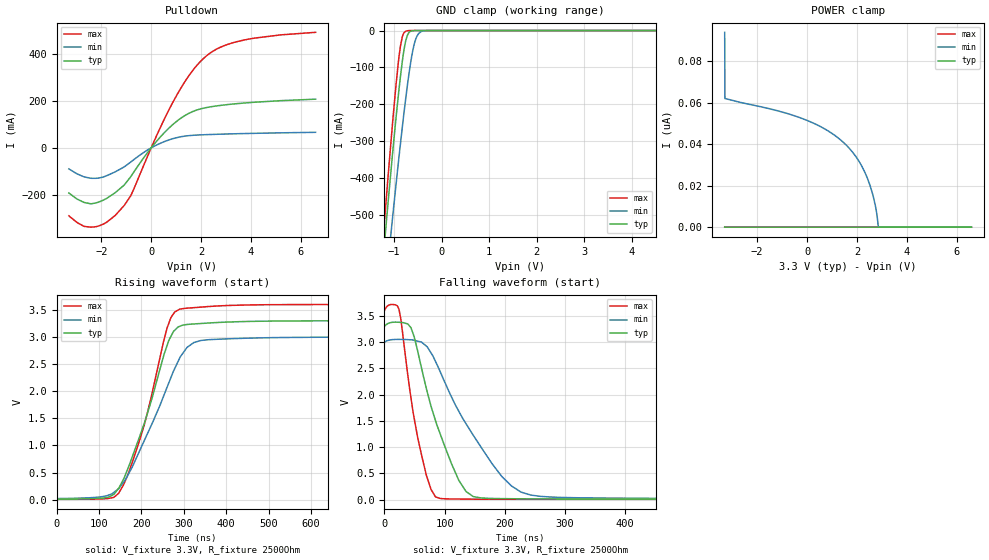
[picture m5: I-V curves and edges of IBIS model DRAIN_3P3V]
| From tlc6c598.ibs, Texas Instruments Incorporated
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|   Model DRAIN_3P3V
[Model]   DRAIN_3P3V
Model_type   Open_drain
Polarity   Non-Inverting
Vmeas = 1.65
Vref = 3.3
Cref = 15pF
Rref = 2500
|   typ   min   max
|   (nom PVT)   (slow PVT)   (fast PVT)
C_comp   2.311p   1.904p   2.542p
|C_comp (ON state)   2.311p   1.904p   2.542p
|C_comp (Low state)   3.527p   2.893p   3.532p
[Voltage Range]   3.3   3   3.6
[Temperature Range]   27   150   -40
[Pullup Reference]   3.3   3   3.6
[Pulldown Reference]   -0   -0   -0
[Power Clamp Reference]   3.3   3   3.6
[GND Clamp Reference]   -0   -0   -0
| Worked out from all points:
|   slope of the pulldown table from 0 to 0.495 V, typ, clamps not added: 8.07 ohm
|   GND clamp passes 1 mA (typ) near -0.63 V on its own axis
|   falling waveform, V_fixture 3.3V, R_fixture 2500Ohm: 20-80 % time 53.1ns typ, 89.4ns min, 30.9ns max; typ from 3.3 V to 0.01 V
|   rising waveform, V_fixture 3.3V, R_fixture 2500Ohm: 20-80 % time 79.2ns typ, 98.3ns min, 71.1ns max; typ from 0.01 V to 3.3 V
[Pulldown]
|   Voltage   I(typ)   I(min)   I(max)
-3.3V     -193.2mA   -90.12mA   -290.9mA
-2.716V   -232.4mA   -123.1mA   -334.7mA
-2.221V   -235.8mA   -130.4mA   -337.4mA
-1.766V   -215mA     -118.3mA   -317mA
-1.092V   -160.2mA   -82.11mA   -247.9mA
-716.1mV  -106.8mA   -52.09mA   -181.3mA
145.2mV   19.15mA    8.223mA    35.19mA
1.046V    115.6mA    44.26mA    229.4mA
1.719V    157.7mA    54.06mA    338.6mA
2.363V    175.3mA    57.15mA    405.7mA
3.749V    192.1mA    61.25mA    462.1mA
6.59V     208.4mA    66.53mA    494.5mA
[GND Clamp]
|   Voltage   I(typ)   I(min)   I(max)
-3.3V     -3.963A    -3.73A     -4.217A
-1.221V   -608.6mA   -754.4mA   -551.3mA
-1.122V   -464.1mA   -625.3mA   -393mA
-1.033V   -338.6mA   -511.9mA   -256.1mA
-953.7mV  -232.9mA   -413.9mA   -143.3mA
-864.6mV  -125.3mA   -307.8mA   -42.56mA
-815.1mV  -74.66mA   -251.3mA   -13.26mA
-745.8mV  -24.39mA   -176.7mA   -1.562mA
-646.8mV  -1.816mA   -84.85mA   -59.99uA
-567.6mV  -129.7uA   -33.75mA   -4.581uA
-399.3mV  -302.4nA   -1.363mA   0A
6.59V     0A         0A         0A
[POWER Clamp]
|   Voltage   I(typ)   I(min)   I(max)
-3.3V     102.3pA    93.86nA    106.1pA
-3.29V    51.15pA    61.95nA    53.03pA
-369.6mV  0A         53.11nA    0A
561mV     0A         48.31nA    0A
1.343V    0A         42.06nA    0A
1.947V    0A         34.2nA     0A
2.363V    0A         25.22nA    0A
2.531V    0A         19.86nA    0A
2.68V     0A         13.58nA    0A
2.779V    0A         7.782nA    0A
2.868V    0A         0A         0A
6.59V     0A         0A         0A
[Ramp]
R_load = 2500
|   typ   min   max
dV/dt_r   1.97411/7.91943e-08   1.78748/9.83448e-08   2.15648/7.10777e-08
dV/dt_f   1.97412/5.31356e-08   1.78738/8.94386e-08   2.15648/3.09195e-08
[Falling Waveform]
V_fixture = 3.3V
V_fixture_min = 3V
V_fixture_max = 3.6V
R_fixture = 2500Ohm
C_fixture = 0F
|   Time   V(typ)   V(min)   V(max)
0s        3.3V       3V         3.6V
24.26ns   3.377V     3.051V     3.621V
44.04ns   3.274V     3.043V     1.939V
54.94ns   2.841V     3.018V     1.196V
69.89ns   2.103V     2.921V     451.8mV
84.85ns   1.503V     2.63V      51.99mV
135.4ns   155.1mV    1.446V     9.803mV
194.7ns   19.57mV    443.8mV    7.612mV
243.1ns   14.16mV    86.88mV    6.999mV
890ns     9.805mV    20.8mV     5.86mV
[Rising Waveform]
V_fixture = 3.3V
V_fixture_min = 3V
V_fixture_max = 3.6V
R_fixture = 2500Ohm
C_fixture = 0F
|   Time   V(typ)   V(min)   V(max)
0s        9.767mV    20.39mV    5.857mV
111.2ns   30.42mV    60.7mV     15.49mV
145.9ns   206.2mV    198.2mV    113mV
168.4ns   577.2mV    456.1mV    462.4mV
208.4ns   1.444V     1.118V     1.425V
260.6ns   2.846V     2.075V     3.169V
290.1ns   3.197V     2.61V      3.513V
323.7ns   3.241V     2.899V     3.542V
356ns     3.257V     2.95V      3.561V
890ns     3.3V       3V         3.6V
